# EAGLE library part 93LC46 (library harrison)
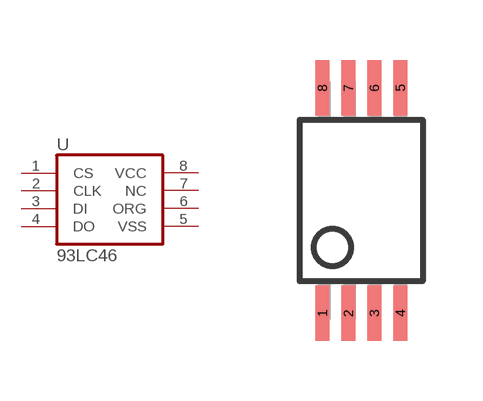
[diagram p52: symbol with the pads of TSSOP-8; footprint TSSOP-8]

Designator prefix U

## 93LC46  [TSSOP-8]
1  CS  in
2  CLK  in
3  DI  in
4  DO  out
5  VSS  pwr
6  ORG  in
7  NC  nc
8  VCC  pwr

## Footprint TSSOP-8 (pad centres in mm)
smd 0.348 x 1.397: 1 -0.973,-2.814; 2 -0.323,-2.815; 3 0.327,-2.815; 4 0.977,-2.815; 5 0.977,2.825; 6 0.327,2.825; 7 -0.323,2.825; 8 -0.973,2.825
